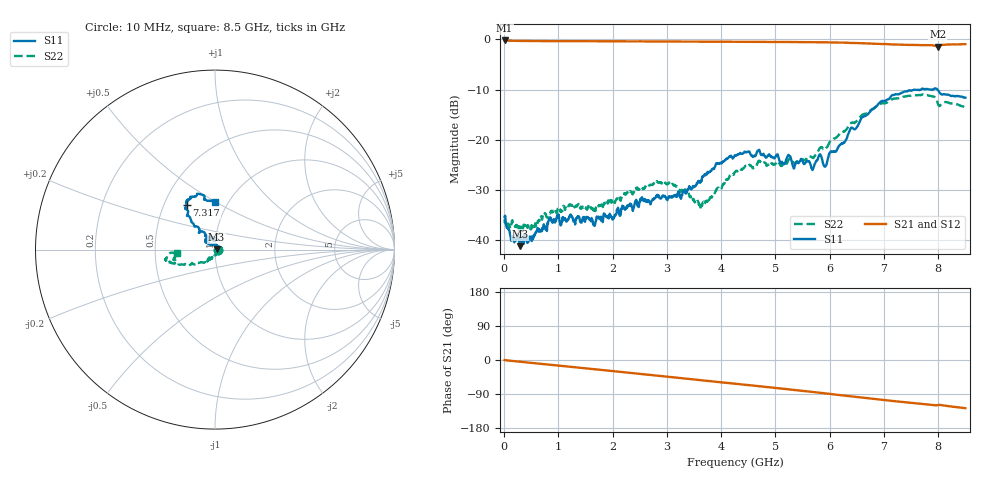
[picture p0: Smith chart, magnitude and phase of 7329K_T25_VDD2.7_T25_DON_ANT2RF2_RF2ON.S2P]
!Agilent Technologies,E5071C,MY46417908,A.11.23
!Date: Mon Aug 31 18:03:06 2020
!Data & Calibration Information:
!Freq	S11:SOLT2(ON)	S21:SOLT2(ON)	S12:SOLT2(ON)	S22:SOLT2(ON)
!PortZ  Port1:50+j0  Port2:50+j0
!Above PortZ is port z conversion or system Z0 setting when saving the data.
!When reading, reference impedance value at option line is always used.
# Hz S dB R 50
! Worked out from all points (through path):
!   1601 points, 10 MHz to 8.5 GHz, reference 50 ohm
!   highest |S21| = -0.20 dB at 10 MHz (marker M1); lowest = -1.4 dB at 7.991 GHz (marker M2)
!   group delay of S21, straight-line fit = 41.8 ps
!   lowest |S11| = -41.1 dB at 291.2 MHz (marker M3), VSWR 1.02, Z = 50.9 + j0.178 ohm
!   |S11| at or under -10 dB: start of sweep to 7.545 GHz; 7.564 GHz to 7.67 GHz (106.1 MHz wide, 1.39 % of centre); 7.988 GHz to end of sweep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
!   |S22| runs from -38.4 to -10.9 dB; largest |S21 - S12| = 0.0047
!   S11 on the Smith chart (normalised r, x): 10 MHz: 1.04, -0.00; 7.317 GHz: 0.65, +0.35; 8.5 GHz: 0.87, +0.49
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1e7  -35.29 -0.5  -0.20 -0.3  -0.20 -0.3  -36.56 -9.6
1.532688e8  -39.18 7.7  -0.26 -2.5  -0.27 -2.5  -35.95 4.3
2.912312e8  -41.13 11.5  -0.28 -4.5  -0.28 -4.6  -38.26 14.0
5.247062e8  -39.56 52.2  -0.31 -7.9  -0.31 -7.9  -37.37 30.9
8.430812e8  -35.57 70.8  -0.33 -12.5  -0.33 -12.5  -34.54 36.4
1.426769e9  -36.46 83.3  -0.35 -20.9  -0.35 -20.9  -33.56 17.9
2.010456e9  -35.39 72.0  -0.36 -29.4  -0.36 -29.4  -32.53 8.7
2.843538e9  -31.26 75.4  -0.38 -41.6  -0.38 -41.6  -28.48 12.9
3.257425e9  -31.67 104.9  -0.39 -47.8  -0.40 -47.7  -30.14 1.5
3.623556e9  -28.36 129.9  -0.41 -53.3  -0.41 -53.3  -33.16 -43.4
4.255e9  -23.03 136.6  -0.46 -62.6  -0.46 -62.6  -26.39 -108.6
4.690112e9  -22.07 126.5  -0.48 -69.0  -0.49 -69.0  -24.14 -118.1
5.14645e9  -24.69 102.8  -0.49 -76.0  -0.49 -76.0  -25.05 -122.5
5.671769e9  -25.79 96.0  -0.54 -84.1  -0.53 -84.1  -23.44 -125.7
5.815038e9  -22.87 99.2  -0.55 -86.3  -0.55 -86.3  -21.63 -125.5
5.921162e9  -25.26 102.7  -0.56 -88.1  -0.55 -88.1  -21.81 -131.7
6.388112e9  -17.72 128.9  -0.69 -95.8  -0.70 -95.8  -16.65 -146.3
7.088538e9  -11.85 126.1  -0.94 -107.2  -0.94 -107.3  -12.35 -161.5
7.316706e9  -10.65 122.4  -1.03 -110.4  -1.03 -110.4  -11.55 -164.5
7.757125e9  -9.93 114.5  -1.13 -116.5  -1.15 -116.5  -10.97 -168.9
7.9906e9  -10.04 103.5  -1.41 -119.1  -1.42 -119.1  -12.73 -175.5
8.5e9  -11.58 89.9  -0.93 -127.2  -0.93 -127.5  -13.40 -175.2
